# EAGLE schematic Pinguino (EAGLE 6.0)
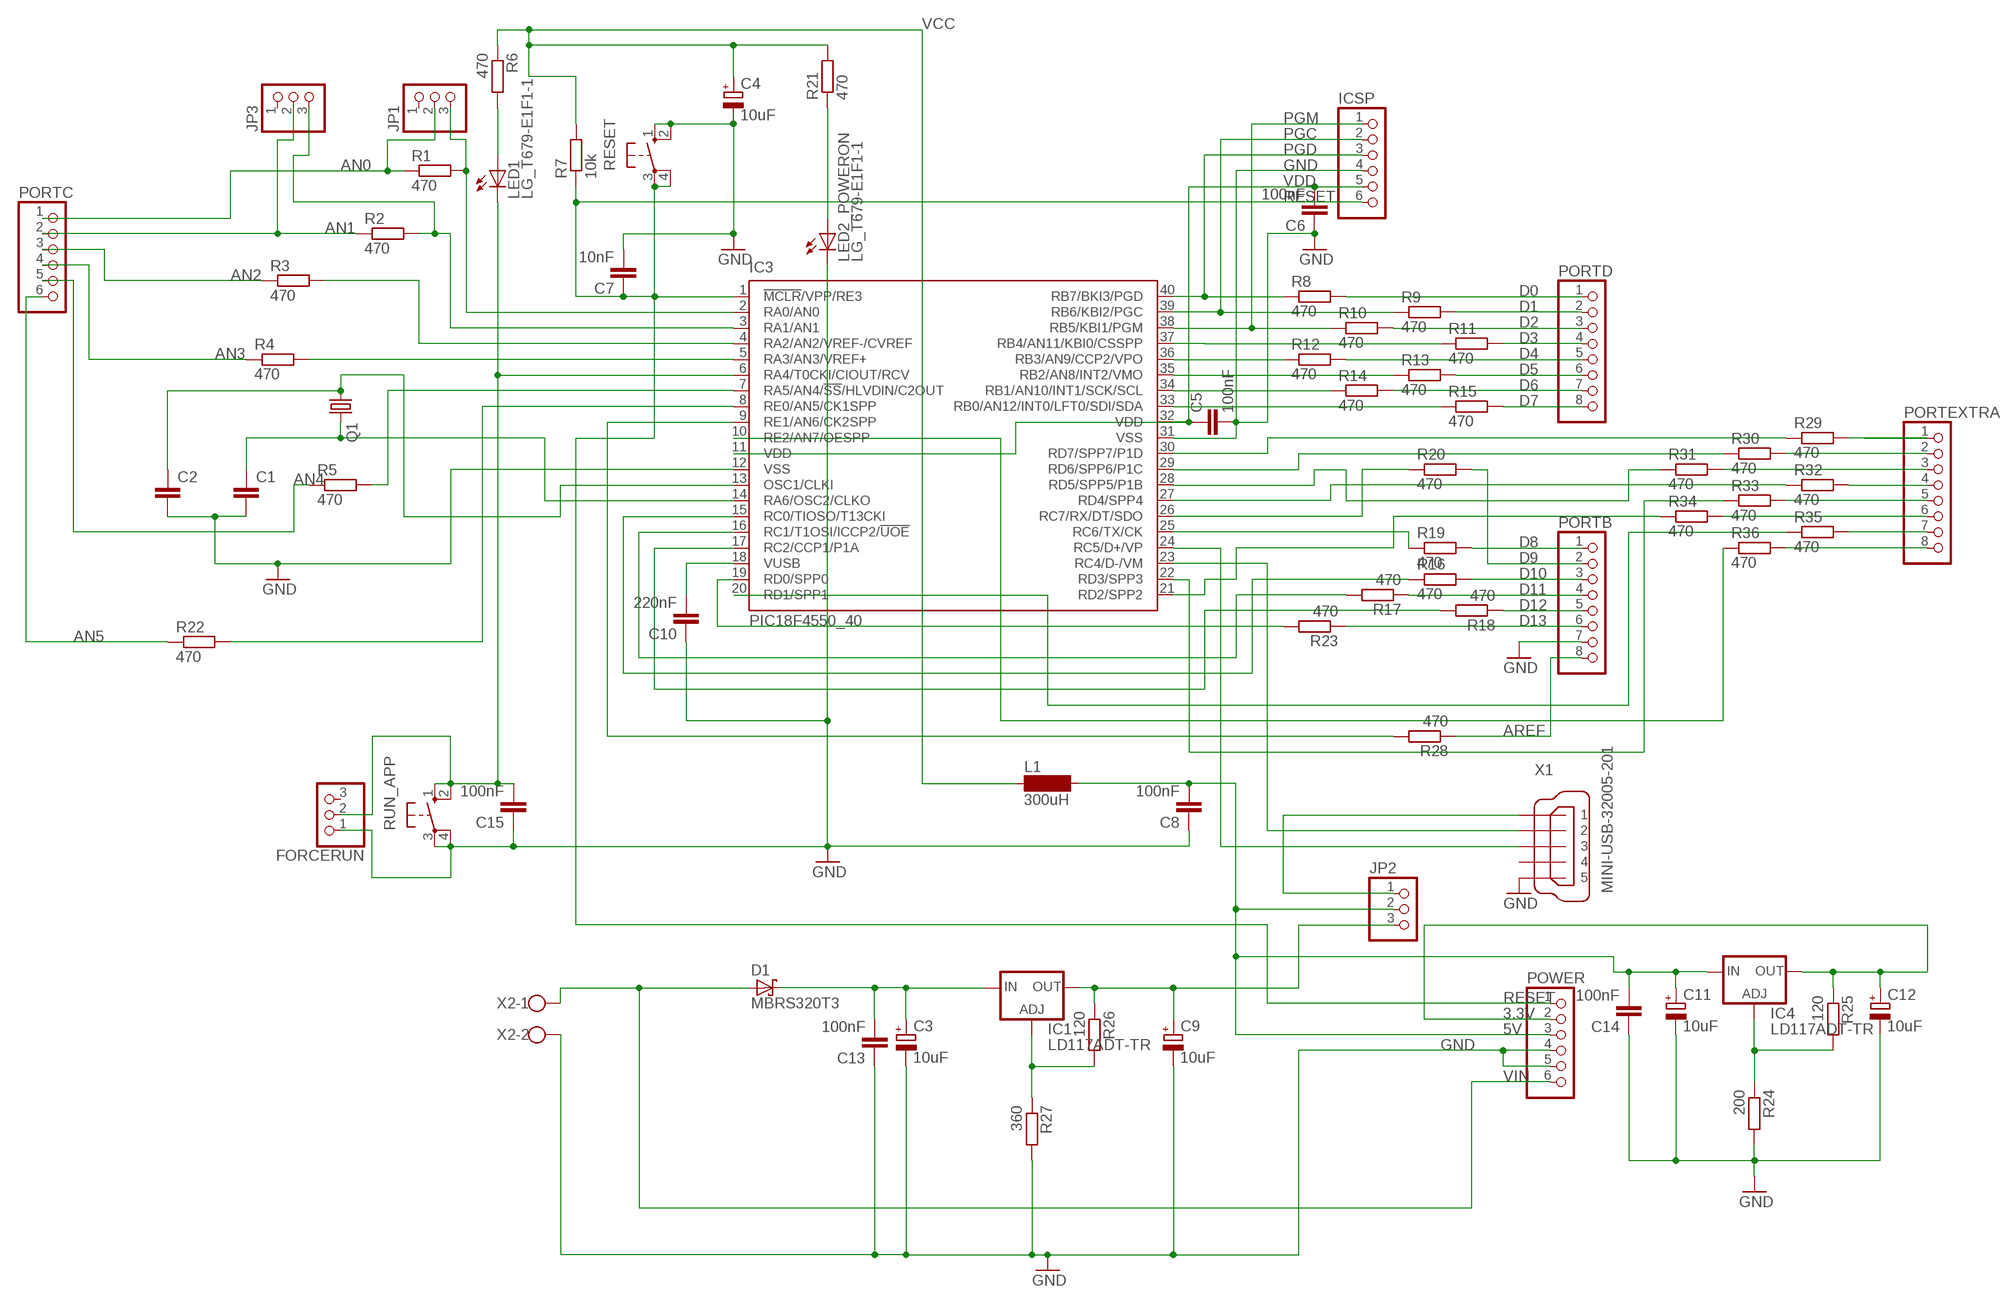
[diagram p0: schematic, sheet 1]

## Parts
C1  C-EUC0603  [C0603]
C2  C-EUC0603  [C0603]
C3  10uF  CPOL-EU153CLV-0505  [153CLV-0505]
C4  10uF  CPOL-EU153CLV-0505  [153CLV-0505]
C5  100nF  C-EUC1206  [C1206]
C6  100nF  C-EUC1206  [C1206]
C7  10nF  C-EUC1206  [C1206]
C8  100nF  C-EUC1206  [C1206]
C9  10uF  CPOL-EU153CLV-0505  [153CLV-0505]
C10  220nF  C-EUC1206  [C1206]
C11  10uF  CPOL-EU153CLV-0505  [153CLV-0505]
C12  10uF  CPOL-EU153CLV-0505  [153CLV-0505]
C13  100nF  C-EUC1206  [C1206]
C14  100nF  C-EUC1206  [C1206]
C15  100nF  C-EUC1206  [C1206]
D1  MBRS320T3  [SMC]
FORCERUN  PINHD-1X3  [1X03]
IC1  LD117ADT-TR  [DPACK]
IC3  PIC18F4550_40  [DIL40]
IC4  LD117ADT-TR  [DPACK]
ICSP  PINHD-1X6  [1X06]
JP1  PINHD-1X3  [1X03]
JP2  PINHD-1X3  [1X03]
JP3  PINHD-1X3  [1X03]
L1  300uH  SM-1206  [SM-1206]
LED1  LG_T679-E1F1-1  [PLCC2]
LED2_POWERON  LG_T679-E1F1-1  [PLCC2]
PORTB  PINHD-1X8  [1X08]
PORTC  PINHD-1X6  [1X06]
PORTD  PINHD-1X8  [1X08]
PORTEXTRA  PINHD-1X8  [1X08]
POWER  PINHD-1X6  [1X06]
Q1  CRYSTALHC49UP  [HC49UP]
R1  470  R-EU_R1210  [R1210]
R2  470  R-EU_R1210  [R1210]
R3  470  R-EU_R1210  [R1210]
R4  470  R-EU_R1210  [R1210]
R5  470  R-EU_R1210  [R1210]
R6  470  R-EU_R1210  [R1210]
R7  10k  R-EU_R1210  [R1210]
R8  470  R-EU_R1210  [R1210]
R9  470  R-EU_R1210  [R1210]
R10  470  R-EU_R1210  [R1210]
R11  470  R-EU_R1210  [R1210]
R12  470  R-EU_R1210  [R1210]
R13  470  R-EU_R1210  [R1210]
R14  470  R-EU_R1210  [R1210]
R15  470  R-EU_R1210  [R1210]
R16  470  R-EU_R1210  [R1210]
R17  470  R-EU_R1210  [R1210]
R18  470  R-EU_R1210  [R1210]
R19  470  R-EU_R1210  [R1210]
R20  470  R-EU_R1210  [R1210]
R21  470  R-EU_R1210  [R1210]
R22  470  R-EU_R1210  [R1210]
R23  470  R-EU_R1210  [R1210]
R24  200  R-EU_R1210  [R1210]
R25  120  R-EU_R1210  [R1210]
R26  120  R-EU_R1210  [R1210]
R27  360  R-EU_R1210  [R1210]
R28  470  R-EU_R1210  [R1210]
R29  470  R-EU_R1210  [R1210]
R30  470  R-EU_R1210  [R1210]
R31  470  R-EU_R1210  [R1210]
R32  470  R-EU_R1210  [R1210]
R33  470  R-EU_R1210  [R1210]
R34  470  R-EU_R1210  [R1210]
R35  470  R-EU_R1210  [R1210]
R36  470  R-EU_R1210  [R1210]
RESET  10-XX  [B3F-10XX]
RUN_APP  10-XX  [B3F-10XX]
X1  MINI-USB-32005-201  [32005-201]
X2  W237-102  [W237-102]

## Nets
3.3V: C12.+ IC4.4(OUT) POWER.2 R25.1
5V: C8.2 C11.+ C14.2 IC4.3(IN) JP2.2 L1.2 POWER.3
AN0: JP1.2 PORTC.1 R1.1
AN1: JP3.2 PORTC.2 R2.1
AN2: PORTC.3 R3.1
AN3: PORTC.4 R4.1
AN4: PORTC.5 R5.1
AN5: PORTC.6 R22.1
AREF: PORTB.8 R28.1
D0: PORTD.1 R8.2
D1: PORTD.2 R9.2
D2: PORTD.3 R10.2
D3: PORTD.4 R11.2
D4: PORTD.5 R12.2
D5: PORTD.6 R13.2
D6: PORTD.7 R14.2
D7: PORTD.8 R15.2
D8: PORTB.1 R19.2
D9: PORTB.2 R20.2
D10: PORTB.3 R16.2
D11: PORTB.4 R17.1
D12: PORTB.5 R18.1
D13: PORTB.6 R23.1
GND: C1.2 C2.2 C3.- C4.- C5.2 C6.1 C7.2 C8.1 C9.- C10.1 C11.- C12.- C13.1 C14.1 C15.1 FORCERUN.1 IC3.12(VSS) IC3.31(VSS) ICSP.4 LED2_POWERON.C PORTB.7 POWER.4 POWER.5 R24.2 R27.2 RESET.1(S) RESET.2(S1) RUN_APP.3(P) RUN_APP.4(P1) X1.5 X2.2
N$1: C1.1 IC3.14(RA6/OSC2/CLKO) Q1.2
N$2: C2.1 IC3.13(OSC1/CLKI) Q1.1
N$3: LED1.A R6.2
N$4: C10.2 IC3.18(VUSB)
N$5: IC3.8(RE0/AN5/CK1SPP) R22.2
N$6: IC3.2(RA0/AN0) JP1.3 R1.2
N$7: IC3.3(RA1/AN1) JP3.3 R2.2
N$8: IC3.4(RA2/AN2/VREF-/CVREF) R3.2
N$9: IC3.5(RA3/AN3/VREF+) R4.2
N$10: IC3.7(RA5/AN4/!SS!/HLVDIN/C2OUT) R5.2
N$11: C15.2 FORCERUN.2 IC3.6(RA4/T0CKI/CIOUT/RCV) LED1.C RUN_APP.1(S) RUN_APP.2(S1)
N$12: IC3.25(RC6/TX/CK) R19.1
N$13: IC3.26(RC7/RX/DT/SDO) R20.1
N$14: IC3.15(RC0/TIOSO/T13CKI) R16.1
N$15: JP2.1 X1.1
N$16: IC3.37(RB4/AN11/KBI0/CSSPP) R11.1
N$17: IC3.36(RB3/AN9/CCP2/VPO) R12.1
N$18: IC3.35(RB2/AN8/INT2/VMO) R13.1
N$19: IC3.34(RB1/AN10/INT1/SCK/SCL) R14.1
N$20: IC3.33(RB0/AN12/INT0/LFT0/SDI/SDA) R15.1
N$21: C9.+ IC1.4(OUT) JP2.3 R26.1
N$22: IC3.23(RC4/D-/VM) X1.2
N$23: IC3.24(RC5/D+/VP) X1.3
N$24: C3.+ C13.2 D1.C IC1.3(IN)
N$25: IC4.1(ADJ) R24.1 R25.2
N$26: IC3.16(RC1/T1OSI/ICCP2/!UOE) R17.2
N$27: PORTEXTRA.1 R29.2
N$28: IC3.17(RC2/CCP1/P1A) R18.2
N$29: IC1.1(ADJ) R26.2 R27.1
N$30: LED2_POWERON.A R21.1
N$31: IC3.19(RD0/SPP0) R23.2
N$32: PORTEXTRA.4 R32.2
N$33: PORTEXTRA.3 R31.2
N$34: IC3.9(RE1/AN6/CK2SPP) R28.2
N$35: PORTEXTRA.2 R30.2
N$36: PORTEXTRA.5 R33.2
N$37: PORTEXTRA.6 R34.2
N$38: PORTEXTRA.7 R35.2
N$39: PORTEXTRA.8 R36.2
N$40: IC3.10(RE2/AN7/OESPP) R36.1
N$41: IC3.20(RD1/SPP1) R35.1
N$42: IC3.21(RD2/SPP2) R34.1
N$43: IC3.22(RD3/SPP3) R33.1
N$44: IC3.27(RD4/SPP4) R32.1
N$45: IC3.28(RD5/SPP5/P1B) R31.1
N$46: IC3.29(RD6/SPP6/P1C) R30.1
N$47: IC3.30(RD7/SPP7/P1D) R29.1
PGC: IC3.39(RB6/KBI2/PGC) ICSP.2 R9.1
PGD: IC3.40(RB7/BKI3/PGD) ICSP.3 R8.1
PGM: IC3.38(RB5/KBI1/PGM) ICSP.1 R10.1
RESET: C7.1 IC3.1(!MCLR!/VPP/RE3) ICSP.6 POWER.1 R7.1 RESET.3(P) RESET.4(P1)
VCC: C4.+ L1.1 R6.1 R7.2 R21.2
VDD: C5.1 C6.2 IC3.11(VDD) IC3.32(VDD) ICSP.5
VIN: D1.A POWER.6 X2.1
Unconnected: FORCERUN.3 JP1.1 JP3.1 X1.4

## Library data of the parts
C1 C2 = rcl:C-EU: CAPACITOR, European symbol
C3 C4 C9 C11 C12 = rcl:CPOL-EU: POLARIZED CAPACITOR, European symbol
C5-C8 C10 C13-C15 = resistor:C-EU: CAPACITOR, European symbol
D1 = diode:MBRS3*0T3: SCHOTTKY BARRIER RECTIFIER 3.0 AMPERES 20, 30, 40 VOLT
FORCERUN JP1-JP3 = pinhead:PINHD-1X3: PIN HEADER
IC1 IC4 = v-reg:LD117A?*: Low drop fixed and adjustable positive voltage regulators 1 A Source: http://www.st.com/stonline/products/literature/ds/7194/ld1117axx.pdf
IC3 = microchip:PIC18F4*_40: USB Microcontrollers with nanoWatt Technology High-Performance, Enhanced Flash, 28/40/44-Pin, Source: http://ww1.microchip.com/downloads/en/devicedoc/39632c.pdf; MF: MICROCHIP; MPN: PIC18F4550-I/P; OC_FARNELL: 9321357; OC_NEWARK: 74K8623
ICSP PORTC POWER = pinhead:PINHD-1X6: PIN HEADER
L1 = inductor-neosid:SM-1206: INDUCTOR; OC_FARNELL: unknown; OC_NEWARK: unknown
LED1 LED2_POWERON = led:*_T679-?-1: LC TOPLED® Low Current LED; COLOR: green
PORTB PORTD PORTEXTRA = pinhead:PINHD-1X8: PIN HEADER
Q1 = crystal:CRYSTAL: CRYSTAL; OC_FARNELL: unknown; OC_NEWARK: unknown
R1-R36 = rcl:R-EU_: RESISTOR, European symbol
RESET RUN_APP = switch-omron:10-XX: OMRON SWITCH; MPN: B3F-1000; OC_FARNELL: 176432; OC_NEWARK: 36M3542
X1 = con-cypressindustries:MINI-USB-: MINI USB-B Conector Source: www.cypressindustries.com; OC_FARNELL: unknown; OC_NEWARK: unknown
X2 = con-wago-500:W237-102: WAGO SCREW CLAMP; MPN: 237-102; OC_FARNELL: unknown; OC_NEWARK: 70K9898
